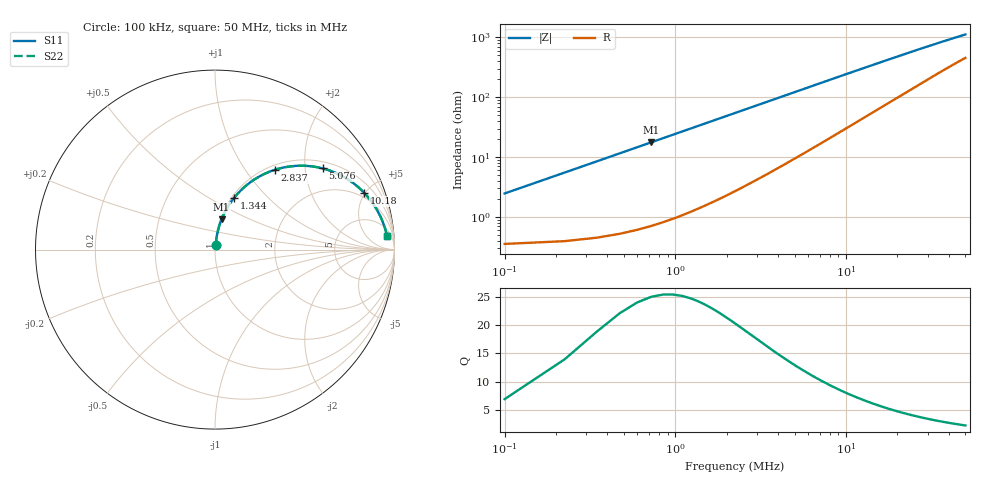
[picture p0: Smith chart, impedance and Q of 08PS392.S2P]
! Coilcraft 0805PS-392 Power Chip Inductor
! 5 February 2003
# MHZ S MA R 50
!Freq  MagS11  AngS11  MagS21  AngS21  MagS12  AngS12  MagS22  AngS22
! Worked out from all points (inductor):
!   403 points, 100 kHz to 50 MHz, reference 50 ohm
!   read as one part in series: L = 3.9 uH near 348.8 kHz
!   highest Q = 24.7 at 722 kHz (marker M1), where L = 3.9 uH
!   S11 on the Smith chart (normalised r, x): 100 kHz: 1.01, +0.05; 1.344 MHz: 1.03, +0.66; 2.837 MHz: 1.08, +1.39; 5.076 MHz: 1.19, +2.48; 10.18 MHz: 1.62, +4.92; 50 MHz: 10, +20
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0.1  0.02467 80.3  0.9962 -1.4  0.9962 -1.4  0.02467 80.3
0.2244  0.05486 82.8  0.9946 -3.1  0.9946 -3.1  0.05486 82.8
0.4732  0.1148 80.8  0.9882 -6.6  0.9882 -6.6  0.1148 80.8
0.5976  0.1443 79.3  0.9835 -8.3  0.9835 -8.3  0.1443 79.3
0.722  0.1733 77.7  0.978 -10.0  0.978 -10.0  0.1733 77.7
0.9708  0.2297 74.5  0.9643 -13.3  0.9643 -13.3  0.2297 74.5
1.344  0.3094 69.6  0.9383 -18.0  0.9383 -18.0  0.3094 69.6
1.5928  0.3587 66.5  0.9181 -21.0  0.9181 -21.0  0.3587 66.5
1.966  0.4266 62.1  0.8848 -25.2  0.8848 -25.2  0.4266 62.1
2.3392  0.4871 58.0  0.8492 -29.1  0.8492 -29.1  0.4871 58.0
2.8368  0.5566 53.1  0.8005 -33.8  0.8005 -33.8  0.5566 53.1
3.832  0.663 44.8  0.7064 -41.4  0.7064 -41.4  0.663 44.8
5.076  0.7509 37.1  0.6045 -48.5  0.6045 -48.5  0.7509 37.1
6.5688  0.8156 30.4  0.508 -54.3  0.508 -54.3  0.8156 30.4
8.4348  0.8629 24.6  0.4193 -59.1  0.4193 -59.1  0.8629 24.6
10.1764  0.8894 20.9  0.3589 -61.9  0.3589 -61.9  0.8894 20.9
13.0376  0.9148 16.6  0.2892 -64.7  0.2892 -64.7  0.9148 16.6
16.7696  0.9323 13.1  0.2303 -66.5  0.2303 -66.5  0.9323 13.1
25.1044  0.9491 8.9  0.1589 -66.9  0.1589 -66.9  0.9491 8.9
33.4392  0.956 6.7  0.1223 -65.6  0.1223 -65.6  0.956 6.7
41.774  0.9597 5.4  0.1002 -63.7  0.1002 -63.7  0.9597 5.4
50  0.962 4.5  0.08582 -61.5  0.08582 -61.5  0.962 4.5
